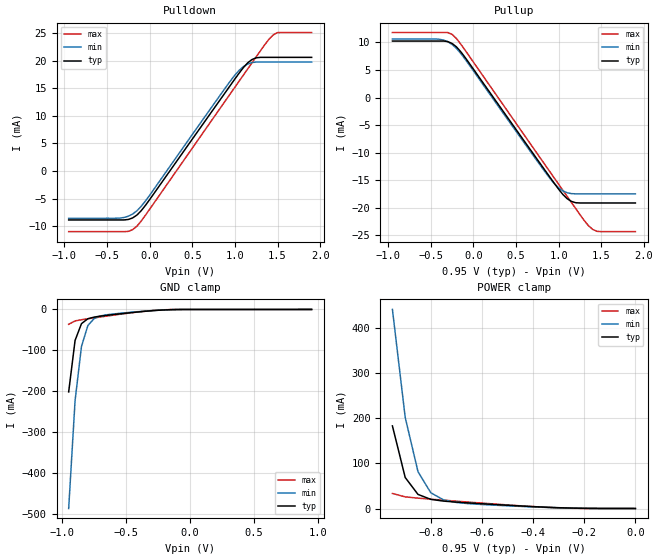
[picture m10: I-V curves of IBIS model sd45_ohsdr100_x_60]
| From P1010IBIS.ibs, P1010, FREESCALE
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[Model] sd45_ohsdr100_x_60
Model_type 3-state
Enable Active-High
Polarity Non-Inverting
|   TYP   MIN   MAX
C_comp   0.00pF   0.00pF   0.00pF
[Model Spec]
Vmeas   0.475   0.425   0.605
[Temperature Range] 65   125   -40
[Voltage Range]   0.95   0.85   1.21
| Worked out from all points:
|   slope of the pulldown table from 0 to 0.142 V, typ, clamps not added: 45.7 ohm
|   slope of the pullup table from 0 to 0.142 V, typ, clamps not added: 45.5 ohm
|   GND clamp passes 1 mA (typ) near -0.19 V on its own axis
|   POWER clamp passes 1 mA (typ) near -0.25 V on its own axis
[Pullup]
|   Vout(V)   TYP   WCS   BCS
-950mV    10.25mA    10.63mA    11.8mA
-400mV    10.25mA    10.58mA    11.8mA
-250mV    9.815mA    9.637mA    11.46mA
-100mV    7.328mA    7.022mA    8.649mA
800mV     -12.33mA   -12.61mA   -11.31mA
1V        -16.63mA   -16.39mA   -15.73mA
1.1V      -18.35mA   -17.27mA   -17.94mA
1.15V     -18.84mA   -17.43mA   -19.04mA
1.3V      -19.13mA   -17.47mA   -22.31mA
1.4V      -19.13mA   -17.47mA   -23.93mA
1.5V      -19.13mA   -17.47mA   -24.33mA
1.9V      -19.13mA   -17.47mA   -24.33mA
[Pulldown]
|   Vout(V)   TYP   WCS   BCS
-950mV    -8.881mA   -8.579mA   -11mA
-350mV    -8.881mA   -8.549mA   -11mA
-250mV    -8.795mA   -8.206mA   -10.95mA
-150mV    -8.006mA   -7.229mA   -10.02mA
0V        -5.189mA   -4.405mA   -6.939mA
950mV     15.58mA    16.36mA    14.07mA
1.1V      18.73mA    18.9mA     17.38mA
1.2V      20.18mA    19.62mA    19.58mA
1.25V     20.49mA    19.73mA    20.68mA
1.45V     20.58mA    19.73mA    24.65mA
1.5V      20.58mA    19.73mA    25.06mA
1.9V      20.58mA    19.73mA    25.07mA
[GND Clamp]
|   Vout(V)   TYP   WCS   BCS
-950mV    -201.6mA   -486.5mA   -36.16mA
-900mV    -75.75mA   -222.9mA   -28.05mA
-850mV    -34.66mA   -90.59mA   -25.11mA
-800mV    -22.71mA   -39.37mA   -22.78mA
-750mV    -18.57mA   -21.91mA   -20.52mA
-700mV    -16.25mA   -15.71mA   -18.29mA
-650mV    -14.32mA   -12.88mA   -16.07mA
-400mV    -5.858mA   -5.175mA   -5.911mA
-200mV    -1.108mA   -1.072mA   -756.7uA
950mV     70.01uA    122.9uA    16.34uA
[POWER Clamp]
|   Vout(V)   TYP   WCS   BCS
-950mV    183.5mA    442.2mA    33.41mA
-900mV    68.86mA    202.2mA    25.88mA
-850mV    31.34mA    81.75mA    23.04mA
-800mV    20.35mA    35.06mA    20.76mA
-750mV    16.45mA    19.08mA    18.55mA
-700mV    14.21mA    13.35mA    16.36mA
-650mV    12.35mA    10.71mA    14.18mA
-300mV    1.805mA    1.559mA    1.409mA
0V        0A         0A         0A
[Ramp]
R_load=50.00
dV/dt_r  1.4958e-01/6.4236e-11  1.3455e-01/6.5371e-11  1.9119e-01/6.5914e-11
dV/dt_f  1.4958e-01/6.5678e-11  1.3454e-01/6.7506e-11  1.9120e-01/6.6813e-11
| End [Model] sd45_ohsdr100_x_60
